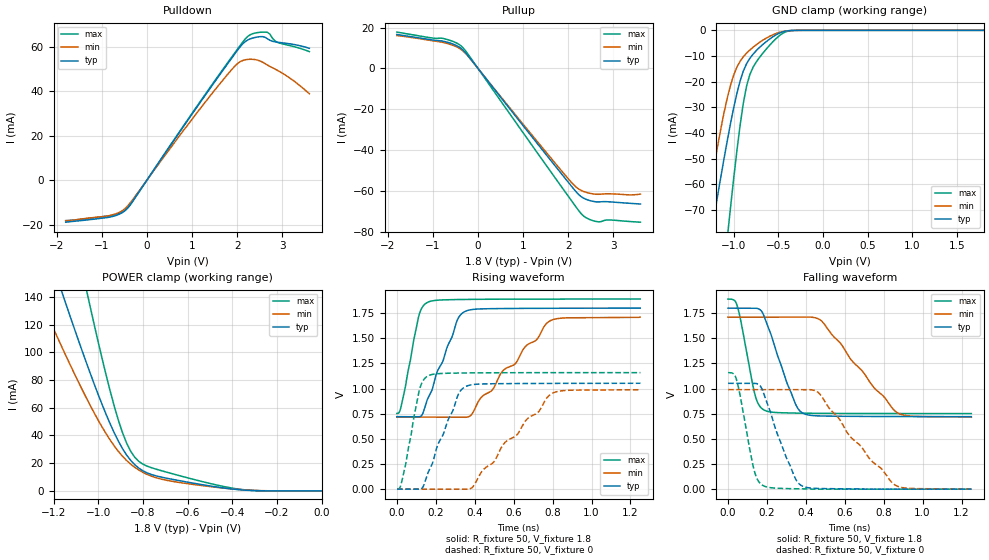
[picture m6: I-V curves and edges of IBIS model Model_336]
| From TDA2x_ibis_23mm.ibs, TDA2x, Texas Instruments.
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| Model based on original model for DDR_SEIOPB_V
|   Sub model SR100_DRV34_1P8
[model]   Model_336
|[Description]  [1.8V-I/O-X-X]
|   , ,
|[Input Load]
|[Output Drive]
|Voltage   1.8V
|Mode   I/O
Model_type   I/O
Polarity   Non-Inverting
Enable   Active-Low
Vinl =  0.775
Vinh =  1.025
Cref =  15.0000pF
Rref =  100.0000M
Vref =  0V
Vmeas =  0.9
C_comp   2p   2p   2p
[Model Spec]
Vinl   0.78   0.735   0.825
Vinh   1.02   0.975   1.065
[Receiver Thresholds]
Tslew_ac = 0.5n
Vth= 0.9
Vth_max= 0.945
Vth_min= 0.81
Vinh_ac= 0.2
Vinh_dc= 0.125
Vinl_ac= -0.2
Vinl_dc= -0.125
[Temperature Range]   25   125   -40
[Voltage Range]   1.8   1.71   1.89
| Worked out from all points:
|   slope of the pulldown table from 0 to 0.27 V, typ, clamps not added: 33.3 ohm
|   slope of the pullup table from 0 to 0.27 V, typ, clamps not added: 35.5 ohm
|   GND clamp passes 1 mA (typ) near -0.48 V on its own axis
|   POWER clamp passes 1 mA (typ) near -0.38 V on its own axis
|   rising waveform, R_fixture 50, V_fixture 1.8: 20-80 % time 126ps typ, 293ps min, 65.7ps max; typ from 0.721 V to 1.8 V
|   rising waveform, R_fixture 50, V_fixture 0: 20-80 % time 126ps typ, 290ps min, 65.5ps max; typ from 0 V to 1.05 V
|   falling waveform, R_fixture 50, V_fixture 1.8: 20-80 % time 117ps typ, 257ps min, 66.4ps max; typ from 1.8 V to 0.721 V
|   falling waveform, R_fixture 50, V_fixture 0: 20-80 % time 120ps typ, 265ps min, 66.1ps max; typ from 1.05 V to 0 V
[POWER_clamp]
-1.8V     464.6mA    344.4mA    740.8mA
-1.273V   197mA      143.3mA    314.4mA
-1.164V   144mA      104.2mA    229mA
-1.145V   135.3mA    97.86mA    215mA
-1.055V   93.25mA    67.59mA    146.5mA
-1.036V   85.18mA    61.89mA    133.3mA
-909.1mV  35.72mA    28.41mA    50.73mA
-872.7mV  25.87mA    21.94mA    34.5mA
-818.2mV  16.45mA    15.08mA    21.33mA
-690.9mV  9.084mA    7.592mA    13.42mA
-400mV    1.38mA     1.43mA     2.039mA
0V        227.3nA    761nA      1.176uA
[Pulldown]
-1.8V     -18.96mA   -18.25mA   -18.29mA
-818.2mV  -16.64mA   -15.93mA   -16.11mA
-600mV    -15.26mA   -14.42mA   -14.86mA
-436.4mV  -12.77mA   -11.85mA   -12.76mA
1.255V    37.14mA    34.14mA    37.53mA
1.855V    54.25mA    49.2mA     54.74mA
2.073V    60.22mA    53.41mA    60.8mA
2.291V    63.64mA    54.44mA    65.5mA
2.618V    64.32mA    52.48mA    66.68mA
2.727V    62.98mA    51.19mA    65.69mA
2.891V    62.13mA    49.45mA    62.08mA
3.6V      59.37mA    38.9mA     57.88mA
[Pullup]
-1.8V     16.66mA    16.14mA    17.84mA
-1.036V   14.05mA    13.69mA    15mA
-763.6mV  13.33mA    12.72mA    14.68mA
-490.9mV  11.4mA     10.78mA    12.65mA
-327.3mV  8.923mA    8.488mA    10.05mA
2.018V    -56.27mA   -54.56mA   -63.19mA
2.182V    -60.67mA   -58.29mA   -68.22mA
2.345V    -63.65mA   -60.35mA   -72.46mA
2.509V    -64.94mA   -61.33mA   -74.33mA
2.673V    -65.44mA   -61.69mA   -75.21mA
2.891V    -65.36mA   -61.45mA   -74.26mA
3.6V      -66.47mA   -61.61mA   -75.37mA
[GND_clamp]
-1.8V     -200.8mA   -187.9mA   -345.9mA
-1.327V   -95.75mA   -76.22mA   -171.1mA
-1.255V   -80.19mA   -60.47mA   -144.9mA
-1.218V   -72.53mA   -52.92mA   -131.9mA
-1.073V   -43.32mA   -26.59mA   -81.54mA
-1.036V   -36.61mA   -21.6mA    -69.55mA
-963.6mV  -24.61mA   -14.37mA   -47.01mA
-854.5mV  -12.98mA   -8.864mA   -21.66mA
-781.8mV  -9.263mA   -6.573mA   -14.36mA
-672.7mV  -5.498mA   -3.827mA   -8.897mA
-345.5mV  -48.81uA   -73.08uA   -79.37uA
1.8V      227.3nA    3.986uA    988nA
[Ramp]
dV/dt_f 0.64800784/0.11717321n 0.59681683/0.25705918n 0.68325122/66.454787p
dV/dt_r 0.63277206/0.12668449n  0.5954817/0.29075118n 0.69633223/65.574612p
R_load = 50
[Rising Waveform]
R_fixture = 50
V_fixture = 1.8
V_fixture_min = 1.71
V_fixture_max = 1.89
0s        720.8mV    716.7mV    752.7mV
22.48ps   720.7mV    716.6mV    825.8mV
114.1ps   719.6mV    716.6mV    1.73V
132.4ps   748.2mV    716.6mV    1.813V
159.6ps   903mV      716.6mV    1.859V
310.5ps   1.68V      716.5mV    1.885V
352.4ps   1.769V     714.7mV    1.886V
383ps     1.785V     739.7mV    1.887V
784.9ps   1.798V     1.671V     1.89V
1.25ns    1.8V       1.71V      1.89V
[Rising Waveform]
R_fixture = 50
V_fixture = 0
V_fixture_min = 0
V_fixture_max = 0
1.313ps   0V         0V         0V
18.78ps   0V         0V         28.98mV
40.61ps   0V         0V         203mV
117.2ps   0V         0V         995.1mV
163ps     176.3mV    0V         1.129V
313.5ps   932mV      0V         1.154V
358ps     1.024V     0V         1.156V
390.8ps   1.04V      24.21mV    1.156V
795.7ps   1.052V     950.2mV    1.158V
1.251ns   1.053V     990.1mV    1.159V
[Falling Waveform]
R_fixture = 50
V_fixture = 1.8
V_fixture_min = 1.71
V_fixture_max = 1.89
0s        1.8V       1.71V      1.89V
46.48ps   1.8V       1.71V      1.83V
138.3ps   1.801V     1.71V      944mV
189.1ps   1.703V     1.71V      783.7mV
306.2ps   1.042V     1.71V      758.1mV
354.7ps   817.3mV    1.71V      756.3mV
386.9ps   753.6mV    1.711V     755.5mV
483.6ps   727.5mV    1.667V     753.8mV
870.7ps   722mV      759.5mV    752mV
1.25ns    720.8mV    716.7mV    751.8mV
[Falling Waveform]
R_fixture = 50
V_fixture = 0
V_fixture_min = 0
V_fixture_max = 0
1.313ps   1.053V     990.1mV    1.159V
42.57ps   1.053V     990.1mV    1.098V
133.2ps   1.053V     990.1mV    199.1mV
183.5ps   953.9mV    990.1mV    32.82mV
296.9ps   327.3mV    990mV      6.053mV
381.9ps   31.28mV    990.4mV    3.003mV
469.2ps   6.723mV    951.7mV    0V
626ps     2.824mV    526.9mV    0V
861.4ps   0V         38.04mV    0V
1.251ns   0V         0V         0V
